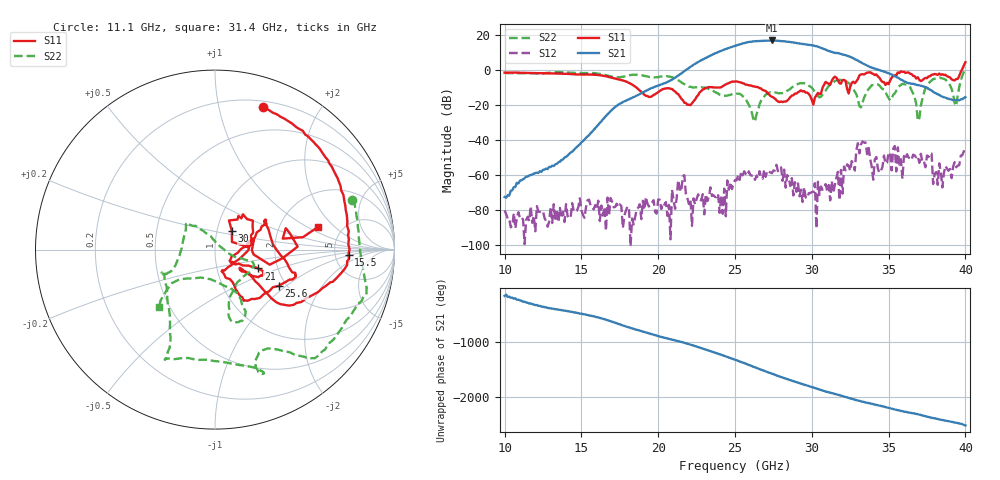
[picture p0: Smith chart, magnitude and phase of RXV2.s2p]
!Keysight Technologies,M9808A,MY58100618,A.14.70.03
!Date: Monday, February 27, 2023 13:44:01
!Correction: S11(Cdelta 2-Port  )
!S21(Cdelta 2-Port  )
!S12(Cdelta 2-Port  )
!S22(Cdelta 2-Port  )
!S2P File: Measurements: S11, S21, S12, S22:
# Hz S  RI  R 50
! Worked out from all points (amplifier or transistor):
!   301 points, 10 GHz to 40 GHz, reference 50 ohm
!   highest |S21| = 16.9 dB at 27.4 GHz (marker M1)
!   |S21| within 3 dB of that: 25.03 GHz to 30.14 GHz (5.108 GHz wide, 18.5 % of centre)
!   unconditionally stable (mu >= 1): start of sweep to 39.73 GHz
!   at 15 GHz: K = 81085.38, MAG = -32.7 dB, |S12| = -80.1 dB
!   at 25 GHz: K = 104.21, MAG = 15.1 dB, |S12| = -62.8 dB
!   at 40 GHz: K = 524.27, MSG = 16.3 dB, |S12| = -47.9 dB
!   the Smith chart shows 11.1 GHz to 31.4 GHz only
!   S11 on the Smith chart (normalised r, x): 11.1 GHz: 0.25, +1.36; 15.5 GHz: 6.71, -0.92; 21 GHz: 1.58, -0.36; 25.6 GHz: 1.83, -0.88; 30 GHz: 1.18, +0.25; 31.4 GHz: 3.31, +1.27
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1e10  0.0877 0.8436  -0.000223 -8.81e-05  -9.81e-05 -1.76e-05  0.6916 0.4546
1.11e10  0.2677 0.7957  -0.000277 0.000654  -6.08e-05 -1.52e-05  0.7646 0.2764
1.5e10  0.7411 0.0812  -0.00487 -0.00714  5.22e-06 -9.92e-05  0.6585 -0.5031
1.55e10  0.7442 -0.0305  -0.0125 -0.00617  4.99e-05 0.000194  0.5836 -0.5826
2e10  0.1889 -0.1375  -0.3587 -0.0454  0.000144 0.000144  -0.1803 -0.6043
2.1e10  0.2407 -0.105  -0.2573 0.5066  -0.000195 1.03e-05  -0.2525 -0.5462
2.27e10  0.2213 0.0653  1.672 -0.6916  0.000142 -0.000153  -0.298 -0.1293
2.37e10  0.2874 0.1345  -1.29 -2.701  -0.000158 0.000179  -0.2201 -0.0875
2.5e10  0.4477 -0.1422  -2.227 4.385  0.000105 0.000717  -0.1617 0.1428
2.56e10  0.3556 -0.2016  3.412 4.843  0.000937 0.000885  -0.1073 0.1321
2.63e10  0.1829 -0.2848  6.163 -2.599  0.000703 0.000207  0.0293 0.017
2.69e10  0.1234 -0.2314  0.3208 -6.933  0.00128 0.000632  0.1673 -0.0566
2.74e10  0.0662 -0.1597  -5.285 -4.631  0.00106 0.000398  0.2172 -0.0929
2.8e10  0.0522 -0.1166  -6.351 2.306  0.00164 0.000324  0.1434 -0.1677
2.86e10  0.1686 -0.021  -1.337 6.181  0.000283 -0.0004  0.0791 -0.2774
2.94e10  0.1788 0.1697  4.781 2.849  0.000168 -3.62e-05  0.1394 -0.3978
3e10  0.0938 0.1049  4.721 -2.011  -8.73e-05 0.000317  0.1447 -0.2793
3.05e10  0.205 -0.00271  1.552 -4.222  -0.000273 -9.98e-06  -0.0257 -0.165
3.14e10  0.5733 0.1257  -2.531 -1.992  4.49e-05 0.000312  -0.3122 -0.3212
3.27e10  0.4524 -0.1208  -0.883 2.006  -0.00178 0.00107  0.0028 -0.2937
3.5e10  0.3527 -0.1877  0.5804 -0.5641  -0.00403 0.00182  -0.00639 -0.1596
4e10  0.6274 -1.562  0.1688 -0.0122  0.00134 0.00377  0.5932 -1.017
